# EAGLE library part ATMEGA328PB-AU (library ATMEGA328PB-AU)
ATMEL - ATMEGA328PB-AU - MCU, 8BIT, ATMEGA, 20MHZ, TQFP-32 Source: Datasheet
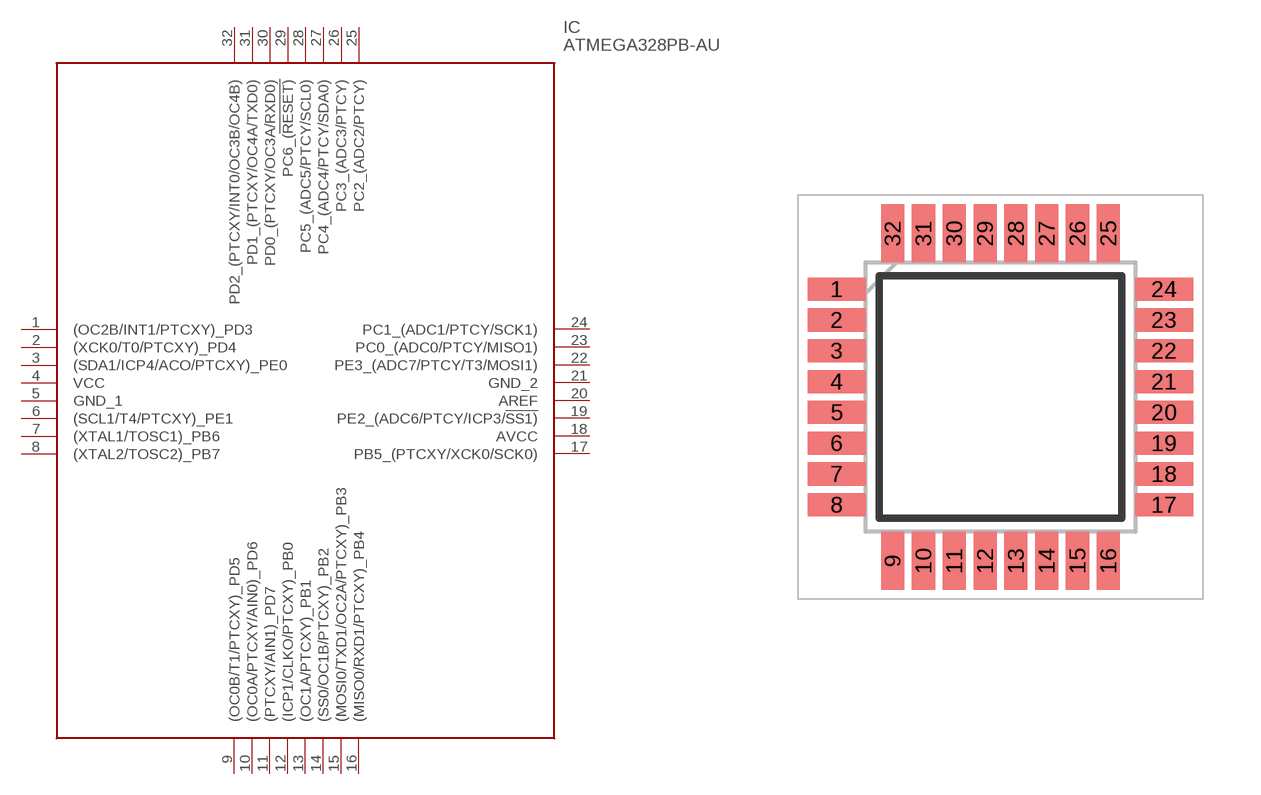
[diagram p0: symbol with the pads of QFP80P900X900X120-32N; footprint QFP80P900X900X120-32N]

Designator prefix IC

## ATMEGA328PB-AU (Description: ATMEL - ATMEGA328PB-AU - MCU, 8BIT, ATMEGA, 20MHZ, TQFP-32; Height: 1.2mm; Manufacturer_Name: Microchip; Manufacturer_Part_Number: ATMEGA328PB-AU; Mouser_Part_Number: 556-ATMEGA328PB-AU; Mouser_Price-Stock: https://www.mouser.com/Search/Refine.aspx?Keyword=556-ATMEGA328PB-AU; RS_Part_Number: 1468928P; RS_Price-Stock: http://uk.rs-online.com/web/p/products/1468928P)  [QFP80P900X900X120-32N]
1  (OC2B/INT1/PTCXY)_PD3
2  (XCK0/T0/PTCXY)_PD4
3  (SDA1/ICP4/ACO/PTCXY)_PE0
4  VCC
5  GND_1
6  (SCL1/T4/PTCXY)_PE1
7  (XTAL1/TOSC1)_PB6
8  (XTAL2/TOSC2)_PB7
9  (OC0B/T1/PTCXY)_PD5
10  (OC0A/PTCXY/AIN0)_PD6
11  (PTCXY/AIN1)_PD7
12  (ICP1/CLKO/PTCXY)_PB0
13  (OC1A/PTCXY)_PB1
14  (SS0/OC1B/PTCXY)_PB2
15  (MOSI0/TXD1/OC2A/PTCXY)_PB3
16  (MISO0/RXD1/PTCXY)_PB4
17  PB5_(PTCXY/XCK0/SCK0)
18  AVCC
19  PE2_(ADC6/PTCY/ICP3/!SS1)
20  AREF
21  GND_2
22  PE3_(ADC7/PTCY/T3/MOSI1)
23  PC0_(ADC0/PTCY/MISO1)
24  PC1_(ADC1/PTCY/SCK1)
25  PC2_(ADC2/PTCY)
26  PC3_(ADC3/PTCY)
27  PC4_(ADC4/PTCY/SDA0)
28  PC5_(ADC5/PTCY/SCL0)
29  PC6_(!RESET)
30  PD0_(PTCXY/OC3A/RXD0)
31  PD1_(PTCXY/OC4A/TXD0)
32  PD2_(PTCXY/INT0/OC3B/OC4B)

## Footprint QFP80P900X900X120-32N (pad centres in mm)
TQFP 32A
smd 1.5 x 0.6: 1 -4.25,2.8; 2 -4.25,2; 3 -4.25,1.2; 4 -4.25,0.4; 5 -4.25,-0.4; 6 -4.25,-1.2; 7 -4.25,-2; 8 -4.25,-2.8; 17 4.25,-2.8; 18 4.25,-2; 19 4.25,-1.2; 20 4.25,-0.4; 21 4.25,0.4; 22 4.25,1.2; 23 4.25,2; 24 4.25,2.8
smd 0.6 x 1.5: 9 -2.8,-4.25; 10 -2,-4.25; 11 -1.2,-4.25; 12 -0.4,-4.25; 13 0.4,-4.25; 14 1.2,-4.25; 15 2,-4.25; 16 2.8,-4.25; 25 2.8,4.25; 26 2,4.25; 27 1.2,4.25; 28 0.4,4.25; 29 -0.4,4.25; 30 -1.2,4.25; 31 -2,4.25; 32 -2.8,4.25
